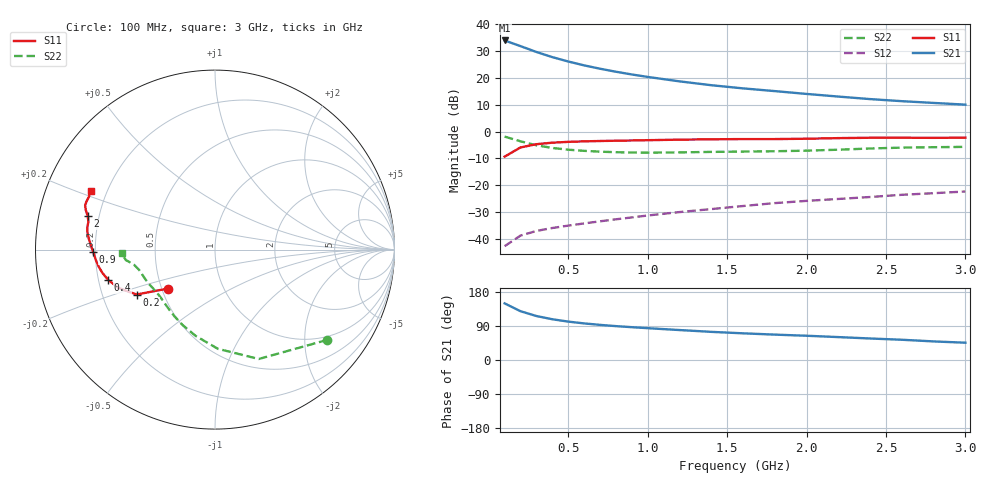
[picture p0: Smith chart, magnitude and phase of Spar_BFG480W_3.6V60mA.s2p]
! Filename: 3_660BFG480.001
! Title: BFG480W
! Bias: Vce=3.6V; Ic=60mA
! Company: NXP Semiconductors NL
! User: Quality&Reliability T&D
! Measure time: 10 Nov 1999 / 12:00:10
#  MHz  S  MA  R 50
! Freq  S11  S21  S12  S22  :
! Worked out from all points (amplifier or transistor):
!   20 points, 100 MHz to 3 GHz, reference 50 ohm
!   highest |S21| = 34.0 dB at 100 MHz (marker M1)
!   |S21| within 3 dB of that: start of sweep to 240.3 MHz
!   unconditionally stable (mu >= 1): 883.1 MHz to end of sweep
!   at 400 MHz: K = 0.69, MSG = 31.9 dB, |S12| = -36.1 dB
!   at 1.2 GHz: K = 1.06, MAG = 23.0 dB, |S12| = -30.1 dB
!   at 3 GHz: K = 1.06, MAG = 14.8 dB, |S12| = -22.4 dB
!   S11 on the Smith chart (normalised r, x): 100 MHz: 0.54, -0.26; 200 MHz: 0.35, -0.24; 400 MHz: 0.24, -0.13; 900 MHz: 0.19, -0.01; 2 GHz: 0.16, +0.13; 3 GHz: 0.14, +0.22
100  0.3393 -140.3  50.26 149.4  0.007203 67.8  0.8031 -38.8
200  0.5034 -150.2  39.36 128.8  0.01135 57.7  0.6563 -68.2
300  0.5794 -158.4  30.63 116.0  0.01387 54.7  0.5531 -88.3
400  0.6181 -164.1  24.55 107.5  0.01574 55.1  0.4929 -102.6
500  0.6407 -168.3  20.33 101.3  0.01743 56.6  0.4573 -113.2
600  0.6547 -171.6  17.22 96.6  0.01916 58.6  0.4352 -121.2
700  0.6644 -174.4  14.91 92.7  0.02097 60.6  0.4203 -127.5
800  0.6723 -176.9  13.09 89.4  0.02287 62.6  0.4104 -132.8
900  0.68 -179.1  11.64 86.6  0.0248 64.6  0.4046 -137.3
1000  0.6882 178.9  10.47 84.0  0.02695 66.1  0.4026 -141.4
1200  0.7038 175.5  8.654 79.1  0.03122 68.5  0.407 -148.0
1400  0.7155 172.9  7.334 74.3  0.0355 70.1  0.4157 -153.0
1600  0.7221 170.4  6.397 70.4  0.04053 71.5  0.4214 -156.8
1800  0.7221 167.7  5.688 67.0  0.04593 72.6  0.4279 -160.7
2000  0.7327 165.3  5.036 64.0  0.05057 73.5  0.4384 -165.2
2200  0.7522 163.1  4.496 60.5  0.05492 73.8  0.4571 -169.1
2400  0.7643 161.2  4.032 56.8  0.05971 73.6  0.4813 -171.7
2600  0.7647 159.5  3.687 53.4  0.06569 73.1  0.5 -173.3
2800  0.7614 157.3  3.419 49.0  0.07036 72.0  0.5089 -175.2
3000  0.7663 154.6  3.175 45.6  0.07569 71.4  0.5163 -178.2
